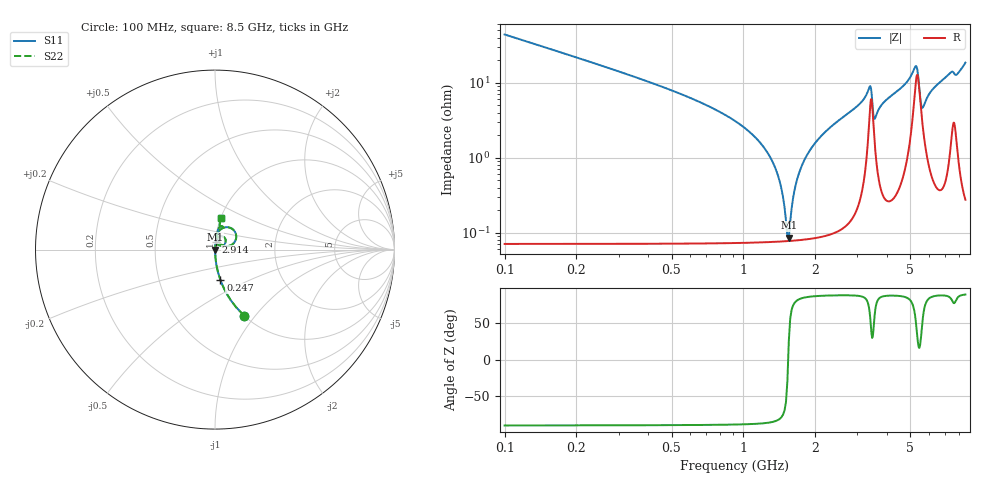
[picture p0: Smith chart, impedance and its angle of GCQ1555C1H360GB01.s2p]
!Murata Part Number: GCQ1555C1H360GB01
!These Parameters are Measured in Series Mode Connection
!Data Generated on Jan 08, 2026
!  o--ll--o
!Port1  Port2
!  o------o
!Operation Temp=25[degC], DC Bias Voltage=0[V]
!Freq. Start=100[MHz] Stop=9[GHz] 401[Steps]
# Hz S RI R 50
!Freq.(Hz) S11(Real) S11(Imag) S21(Real) S21(Imag) S12(Real) S12(Imag) S22(Real) S22(Imag)
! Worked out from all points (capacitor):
!   401 points, 100 MHz to 8.5 GHz, reference 50 ohm
!   read as one part in series: C = 36 pF near 142 MHz
!   lowest |Z| = 86.1 mohm at 1.549 GHz (marker M1)
!   series resonance near 1.539 GHz, so ESL is about 300 pH
!   S11 on the Smith chart (normalised r, x): 100 MHz: 1.00, -0.88; 247 MHz: 1.00, -0.35; 2.914 GHz: 1.00, +0.09; 8.5 GHz: 1.01, +0.37
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1e8  0.1628 -0.3683  0.8372 0.3683  0.8372 0.3683  0.1628 -0.3683
2.47e8  0.0302 -0.1691  0.9698 0.1691  0.9698 0.1691  0.0302 -0.1691
1.234e9  0.000915 -0.0129  0.9991 0.0129  0.9991 0.0129  0.000915 -0.0129
1.402e9  0.000791 -0.00545  0.9992 0.00545  0.9992 0.00545  0.000791 -0.00545
1.507e9  0.000773 -0.00124  0.9992 0.00124  0.9992 0.00124  0.000773 -0.00124
1.549e9  0.000776 0.000371  0.9992 -0.000371  0.9992 -0.000371  0.000776 0.000371
1.696e9  0.000827 0.00572  0.9992 -0.00572  0.9992 -0.00572  0.000827 0.00572
1.906e9  0.000993 0.0128  0.999 -0.0128  0.999 -0.0128  0.000993 0.0128
2.284e9  0.00154 0.0246  0.9985 -0.0246  0.9985 -0.0246  0.00154 0.0246
2.914e9  0.00376 0.0451  0.9962 -0.0451  0.9962 -0.0451  0.00376 0.0451
3.376e9  0.0413 0.0741  0.9587 -0.0741  0.9587 -0.0741  0.0413 0.0741
3.544e9  0.0165 0.0279  0.9835 -0.0279  0.9835 -0.0279  0.0165 0.0279
3.817e9  0.00595 0.0516  0.994 -0.0516  0.994 -0.0516  0.00595 0.0516
4.3e9  0.00822 0.072  0.9918 -0.072  0.9918 -0.072  0.00822 0.072
5.266e9  0.1034 0.1093  0.8966 -0.1093  0.8966 -0.1093  0.1034 0.1093
5.371e9  0.1119 0.0461  0.8881 -0.0461  0.8881 -0.0461  0.1119 0.0461
5.56e9  0.0389 0.0268  0.9611 -0.0268  0.9611 -0.0268  0.0389 0.0268
5.707e9  0.0203 0.0454  0.9797 -0.0454  0.9797 -0.0454  0.0203 0.0454
6.169e9  0.0116 0.0788  0.9884 -0.0788  0.9884 -0.0788  0.0116 0.0788
7.114e9  0.0204 0.1193  0.9796 -0.1193  0.9796 -0.1193  0.0204 0.1193
7.807e9  0.0311 0.1213  0.9689 -0.1213  0.9689 -0.1213  0.0311 0.1213
8.5e9  0.0357 0.1782  0.9643 -0.1782  0.9643 -0.1782  0.0357 0.1782
